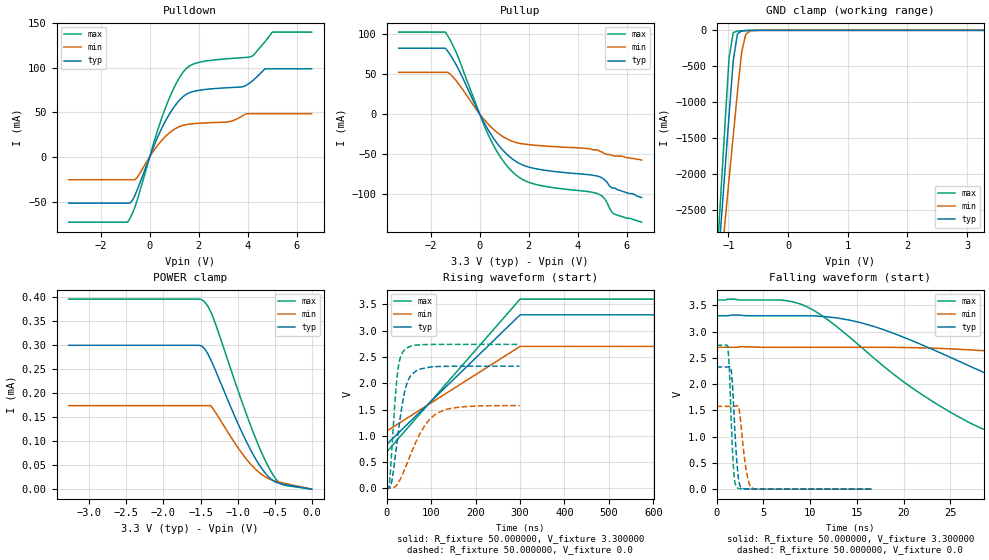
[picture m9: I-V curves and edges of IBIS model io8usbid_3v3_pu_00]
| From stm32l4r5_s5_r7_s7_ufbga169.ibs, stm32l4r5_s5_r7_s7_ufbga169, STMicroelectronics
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|   Model io8usbid_3v3_pu_00
[Model]  io8usbid_3v3_pu_00
Model_type I/O
Polarity   Non-Inverting
Enable   Active-Low
Vinl =   0.990000V
Vinh =   2.310000V
Vmeas =  1.650000V
Cref =   100.000000nF
Rref =   1.000000k
Vref =   3.300000V
C_comp   2.116400pF   2.092700pF   2.152900pF
[Temperature Range]   25.000000   0.125000k   -40.000000
[Pullup Reference]   3.300000V   2.700000V   3.600000V
[Pulldown Reference]   0.0V   0.0V   0.0V
[POWER Clamp Reference]   3.300000V   2.700000V   3.600000V
[GND Clamp Reference]   0.0V   0.0V   0.0V
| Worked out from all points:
|   slope of the pulldown table from 0 to 0.495 V, typ, clamps not added: 15.4 ohm
|   slope of the pullup table from 0 to 0.495 V, typ, clamps not added: 18.1 ohm
|   GND clamp passes 1 mA (typ) near -0.59 V on its own axis
|   rising waveform, R_fixture 50.000000, V_fixture 3.300000: 20-80 % time 180ns typ, 180ns min, 180ns max; typ from 0.836 V to 3.3 V
|   rising waveform, R_fixture 50.000000, V_fixture 0.0: 20-80 % time 23.9ns typ, 53.3ns min, 14.3ns max; typ from 0.001 V to 2.33 V
|   falling waveform, R_fixture 50.000000, V_fixture 3.300000: 20-80 % time 21ns typ, 41.6ns min, 13.6ns max; typ from 3.3 V to 0.836 V
|   falling waveform, R_fixture 50.000000, V_fixture 0.0: 20-80 % time 449ps typ, 626ps min, 371ps max; typ from 2.33 V to 0.001 V
[Pulldown]
|Voltage   I(typ)   I(min)   I(max)
-3.3V     -51.63mA   -25.53mA   -73.04mA
-900mV    -51.63mA   -25.53mA   -73.04mA
-500mV    -36.51mA   -22.79mA   -47.71mA
200mV     14.02mA    8.316mA    18.9mA
700mV     42.98mA    24.4mA     58.9mA
1.2V      63.06mA    33.8mA     88.14mA
1.6V      71.63mA    36.67mA    101.4mA
3.2V      77.51mA    39.29mA    110mA
4.1V      83.28mA    48.38mA    112mA
4.7V      98.63mA    48.38mA    129mA
5V        98.63mA    48.38mA    139.8mA
6.6V      98.63mA    48.43mA    139.8mA
[Pullup]
|Voltage   I(typ)   I(min)   I(max)
-3.3V     82.69mA    52.35mA    102.9mA
-1.4V     82.69mA    52.35mA    102.9mA
-900mV    58.56mA    39.63mA    73.37mA
100mV     -6.166mA   -3.962mA   -8.038mA
500mV     -27.53mA   -17.49mA   -35.6mA
1V        -47.29mA   -29.37mA   -60.81mA
1.5V      -60.05mA   -35.95mA   -77.15mA
2.4V      -69.45mA   -39.66mA   -89.34mA
4.8V      -78.1mA    -45mA      -100.1mA
5.1V      -83mA      -50mA      -106.7mA
5.5V      -93mA      -53mA      -126mA
6.6V      -105mA     -58mA      -136mA
[GND_clamp]
|Voltage   I(typ)   I(min)   I(max)
-3.3V     -9.914A    -9.595A    -9.188A
-1.2V     -3.541A    -3.911A    -3.279A
-1.13V    -2.75A     -3.295A    -2.301A
-1.06V    -1.963A    -2.68A     -1.33A
-990mV    -1.183A    -2.069A    -386.7mA
-920mV    -424.7mA   -1.463A    -31.42mA
-850mV    -49.12mA   -868.7mA   -10.48mA
-780mV    -9.121mA   -308.3mA   -6.715mA
-710mV    -3.648mA   -53.81mA   -3.986mA
-640mV    -1.726mA   -11.03mA   -1.885mA
-430mV    -22.46uA   -116.8uA   -9.748uA
3.28V     0A         0A         0A
[POWER_clamp]
|Voltage   I(typ)   I(min)   I(max)
-3.28V    299.3uA    173.7uA    395.4uA
-1.48V    297.5uA    173.7uA    393.9uA
-1.4V     281.3uA    173.7uA    380.3uA
-1.36V    268.9uA    173.7uA    368.3uA
-1.32V    255uA      164.8uA    353.1uA
-1.04V    152.4uA    96.77uA    226.2uA
-880mV    98.76uA    62.4uA     155.8uA
-720mV    53.77uA    36.12uA    92.05uA
-560mV    22.58uA    20.52uA    39.82uA
-480mV    14.4uA     16.42uA    20.64uA
-400mV    10.72uA    13.39uA    9.937uA
0V        0A         0A         0A
[Ramp]
| variable   typ   min   max
dV/dt_r  1.39450/23.89300n   0.94482/53.26837n   1.64288/14.28860n
dV/dt_f  1.47839/21.08553n   0.96684/44.67589n   1.74562/13.58476n
R_load = 50.000000
[Rising Waveform]
R_fixture= 50.000000
V_fixture= 3.300000
V_fixture_min= 2.700000
V_fixture_max= 3.600000
|time   V(typ)   V(min)   V(max)
0s        836mV      1.089V     690.6mV
300.3ns   3.3V       2.7V       3.6V
600.6ns   3.3V       2.7V       3.6V
29.73us   3.3V       2.7V       3.6V
[Rising Waveform]
R_fixture= 50.000000
V_fixture= 0.0
V_fixture_min= 0.0
V_fixture_max= 0.0
|time   V(typ)   V(min)   V(max)
0s        930.6uV    1.396mV    659.7uV
6.607ns   7.941mV    4.351mV    110.5mV
13.21ns   206.2mV    9.431mV    914.9mV
19.22ns   580.8mV    34.44mV    1.677V
25.23ns   994.9mV    89.16mV    2.222V
30.03ns   1.304V     160.4mV    2.459V
40.84ns   1.837V     365.3mV    2.638V
66.07ns   2.232V     882.7mV    2.724V
117.1ns   2.318V     1.443V     2.738V
299.1ns   2.325V     1.576V     2.739V
[Falling Waveform]
R_fixture= 50.000000
V_fixture= 3.300000
V_fixture_min= 2.700000
V_fixture_max= 3.600000
|time   V(typ)   V(min)   V(max)
0s        3.3V       2.7V       3.6V
9.61ns    3.3V       2.7V       3.476V
15.32ns   3.173V     2.7V       2.726V
24.62ns   2.538V     2.673V     1.504V
29.13ns   2.177V     2.627V     1.101V
33.93ns   1.823V     2.554V     903.7mV
44.44ns   1.231V     2.33V      781mV
54.65ns   1.023V     2.075V     737.6mV
90.99ns   869.5mV    1.322V     697.4mV
149.5ns   836mV      1.089V     690.6mV
[Falling Waveform]
R_fixture= 50.000000
V_fixture= 0.0
V_fixture_min= 0.0
V_fixture_max= 0.0
|time   V(typ)   V(min)   V(max)
0s        2.325V     1.576V     2.739V
1.201ns   2.325V     1.576V     2.692V
1.368ns   2.331V     1.576V     2.302V
1.535ns   2.294V     1.576V     1.489V
1.802ns   1.677V     1.576V     442.7mV
2.202ns   453.9mV    1.588V     30mV
2.569ns   46.7mV     1.305V     8.871mV
3.203ns   4.988mV    333.1mV    5.102mV
3.804ns   2.904mV    21.64mV    4.279mV
16.62ns   930.6uV    1.396mV    659.7uV
